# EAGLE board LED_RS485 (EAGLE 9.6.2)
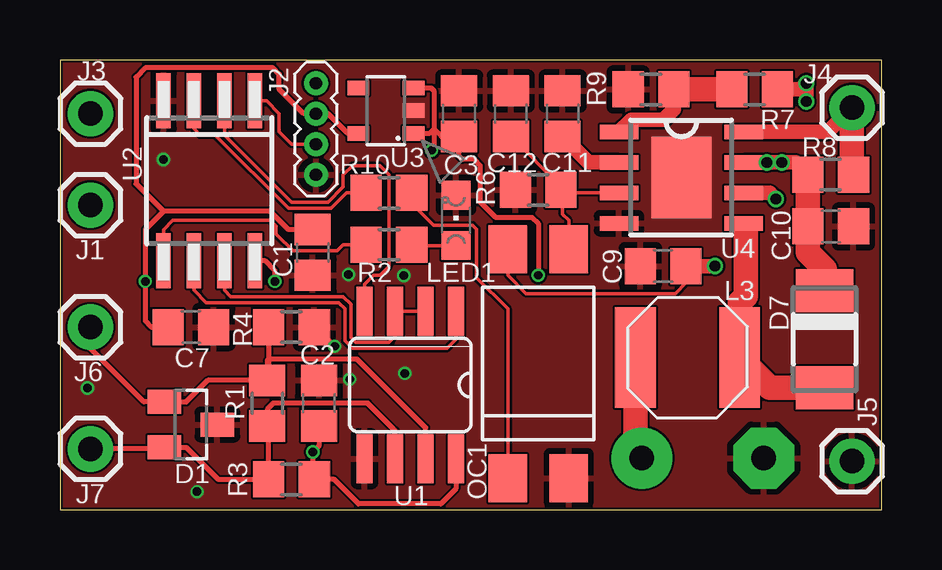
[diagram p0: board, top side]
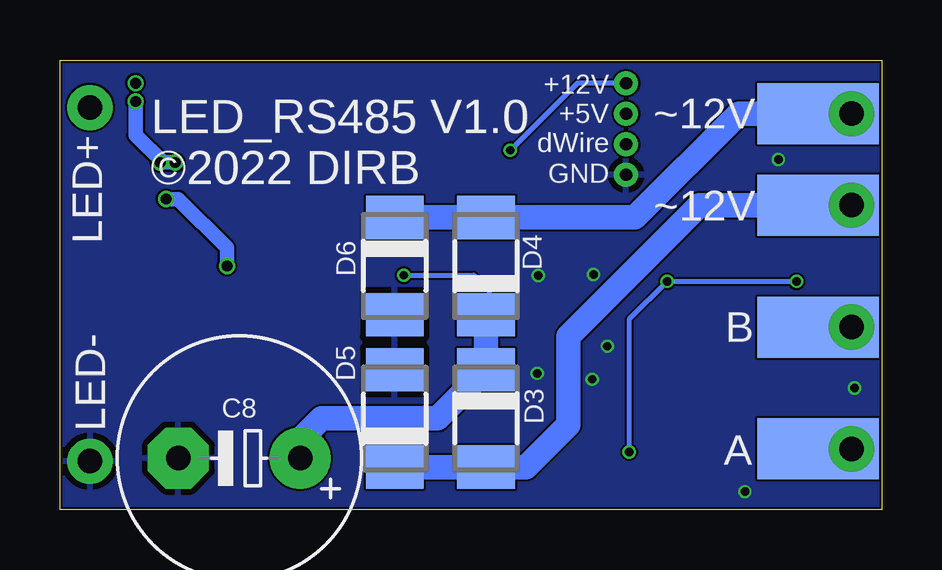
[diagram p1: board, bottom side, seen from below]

Size 34.27 x 18.75 mm. Coordinates in mm from the lower left corner, seen from the top.
Outline: 0,0 34.27,0 34.27,18.75 0,18.75 0,0
Copper layers (1*16): Top 0.035mm / dielectric 0.2mm / Bottom 0.035mm
Design rules "jlcpcb-2-layer": minimum track width 3.5mil, minimum drill 0.2mm, track to track 3.5mil, track to pad 5mil, pad to pad 5mil, via to via 5mil, smd to smd 0mil, copper to edge 0.1mm, drill to drill 5mil, minimum pad ring 4mil, minimum via ring 4mil, stop-mask expansion 3mil, vias tented up to drill 100mil, thermal gap 10mil

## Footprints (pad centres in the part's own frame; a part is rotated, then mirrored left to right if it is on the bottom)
C0805 = smd 1.3 x 1.5: 1 -0.95,0; 2 0.95,0
E5-10,5 = drill 1.016 pad 2.54: + -2.54,0 | drill 1.016 pad 2.54 octagon: - 2.54,0
SOT23 = smd 1 x 1.4: 1 -0.95,-1.1; 2 0.95,-1.1; 3 0,1.1
DO-214AC = smd 1.8 x 2.4: A 2.025,0; C -2.025,0
1X01 = drill 1.016 pad 1.88: 1 0,0
1X04_1.27MM = drill 0.508 pad 1: 1 0,0; 2 1.27,0; 3 2.54,0; 4 3.81,0
L5040S = smd 4.2 x 1.7: 1 0,2.175; 2 0,-2.175
CHIPLED_0805 = smd 1.2 x 1.2: A 0,-1.05; C 0,1.05
DIL4-SMD = smd 1.6 x 2: 1 -1.27,-4.77; 2 1.27,-4.77; 3 1.27,4.77; 4 -1.27,4.77
SMD2,54-5,08 = smd 2.54 x 5.08: 1 0,0
R0805 = smd 1.3 x 1.5: 1 -0.95,0; 2 0.95,0
SO08 = smd 0.66 x 2.032: 1 -1.905,-3.073; 2 -0.635,-3.073; 3 0.635,-3.073; 4 1.905,-3.073; 5 1.905,3.073; 6 0.635,3.073; 7 -0.635,3.073; 8 -1.905,3.073
SOIC8_EIAJ_208MIL = smd 0.6 x 2.286: 1 -1.905,-3.33; 2 -0.635,-3.33; 3 0.635,-3.33; 4 1.905,-3.33; 5 1.905,3.33; 6 0.635,3.33; 7 -0.635,3.33; 8 -1.905,3.33
SOT23-5 = smd 0.9 x 0.6: 1 -1.15,0.95; 2 -1.15,0; 3 -1.15,-0.95; 4 1.15,-0.95; 5 1.15,0.95
SOP8-EP = smd 0.6 x 1.6: 1 -1.905,-2.6; 2 -0.635,-2.6; 3 0.635,-2.6; 4 1.905,-2.6; 5 1.905,2.6; 6 0.635,2.6; 7 -0.635,2.6; 8 -1.905,2.6 | smd 3.4 x 2.5: EP 0,0

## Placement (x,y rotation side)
C1  10u  [C0805]  10.54,10.73 270 top
C2  100n  [C0805]  10.79,4.45 90 top
C3  100n  [C0805]  16.64,16.51 90 top
C7  100n  [C0805]  5.46,7.62 0 top
C8  470u/25V  [E5-10,5]  26.8,2.16 180 bottom
C9  1u  [C0805]  25.15,10.16 180 top
C10  1u  [C0805]  32.13,11.81 0 top
C11  1n  [C0805]  20.95,16.51 90 top
C12  1n  [C0805]  18.8,16.51 270 top
D1  PSM712  [SOT23]  5.46,3.56 270 top
D3  SS14  [DO-214AC]  16.51,3.81 270 bottom
D4  SS14  [DO-214AC]  16.51,10.16 90 bottom
D5  SS14  [DO-214AC]  20.32,3.81 90 bottom
D6  SS14  [DO-214AC]  20.32,10.16 270 bottom
D7  SS14  [DO-214AC]  31.88,7.11 270 top
J1  [1X01]  1.27,12.7 0 top
J2  [1X04_1.27MM]  10.67,13.97 90 top
J3  ~12V  [1X01]  1.27,16.51 0 top
J4  [1X01]  33.02,16.76 0 top
J5  [1X01]  33.02,2.03 0 top
J6  [1X01]  1.27,7.62 0 top
J7  [1X01]  1.27,2.54 0 top
L3  33uH  [L5040S]  26.16,6.35 90 top
LED1  [CHIPLED_0805]  16.51,12.06 0 top
OC1  LTV816S  [DIL4-SMD]  19.94,6.1 0 top
PAD1  ~12V  [SMD2,54-5,08]  2.67,12.7 90 bottom
PAD2  ~12V  [SMD2,54-5,08]  2.67,16.51 270 bottom
PAD5  [SMD2,54-5,08]  2.67,7.62 270 bottom
PAD6  [SMD2,54-5,08]  2.67,2.54 270 bottom
R1  120 (opt)  [R0805]  8.64,4.45 90 top
R2  1K  [R0805]  13.72,11.05 0 top
R3  360 (opt)  [R0805]  9.65,1.27 0 top
R4  360 (opt)  [R0805]  9.65,7.62 180 top
R6  4k7  [R0805]  19.94,13.34 0 top
R7  430k  [R0805]  28.96,17.53 180 top
R8  0R75  [R0805]  32.13,13.97 0 top
R9  10k  [R0805]  24.64,17.53 180 top
R10  1K  [R0805]  13.72,13.21 180 top
U1  MAX485CSA  [SO08]  14.6,5.21 180 top
U2  ATTINY85-20S  [SOIC8_EIAJ_208MIL]  6.22,13.72 180 top
U3  LP2981AIM5-5.0/NOPB  [SOT23-5]  13.59,16.64 180 top
U4  BP1808  [SOP8-EP]  25.91,13.84 270 top

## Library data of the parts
C1-C3 C7-C12 = rcl; SPICEPREFIX: C
D1 D3-D7 = diode
J1-J7 = SparkFun-Connectors
L3 = OPL_Inductor
LED1 = led
OC1 = optocoupler
PAD1 PAD2 PAD5 PAD6 = wirepad
R1-R4 R6-R10 = rcl; SPICEPREFIX: R
U1 = maxim; MPN: MAX3468CSA+; OC_FARNELL: unknown; OC_NEWARK: 76K6721
U2 = _hhn_attiny25_45_85
U3 = Regulators
U4 = BP1808

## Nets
+5V: C1.1 C2.1 C7.1 J2.3 R3.2 U1.8 U2.8 U3.5
A: D1.2 J7.1 PAD6.1 R1.1 R3.1 U1.6
B: D1.1 J6.1 PAD5.1 R1.2 R4.2 U1.7
DIR: U1.2 U1.3 U2.7
GND: C1.2 C2.2 C3.2 C7.2 C8.- C9.2 C10.2 C11.2 C12.1 D1.3 D5.A D6.A J2.1 J5.1 LED1.C OC1.2 R4.1 R6.1 R9.2 U1.5 U2.4 U3.2 U4.4 U4.EP
LED: R2.1 U2.5
N$1: C3.1 C8.+ D3.C D4.C J2.4 L3.1 U3.1 U3.3
N$6: LED1.A R2.2
N$7: R10.2 U2.3
N$10: D3.A D5.C J1.1 PAD1.1
N$11: J2.2 U2.1
N$12: C12.2 OC1.3 R6.2 U4.3
N$14: D4.A D6.C J3.1 PAD2.1
N$15: D7.A L3.2 U4.5
N$18: C9.1 OC1.4 U4.6
N$19: C11.1 U4.2
N$20: C10.1 D7.C R7.1 R8.1 U4.7
N$21: J4.1 R8.2 U4.8
N$23: R7.2 R9.1 U4.1
PWM: OC1.1 R10.1
RXD: U1.1 U2.6
TXD: U1.4 U2.2

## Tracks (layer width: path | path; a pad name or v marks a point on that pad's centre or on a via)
+5V  (via drill 0.35)
  Top 0.2: U3.5 12,15.69 11.18,16.51 J2.3 10.16,16.51 9.14,17.53 9.14,18.16 8.89,18.41 3.56,18.41 3.18,18.03 3.18,13.59 4.32,12.45 | U2.8 8.14,10.4 8.52,10.4 8.95,9.97 v8.95,9.52 | C2.1 10.79,2.67 v10.54,2.41 10.54,1.33 R3.2 11.43,1.27 12.45,0.25 15.87,0.25 16.51,0.89 U1.8 | C1.1 9.53,11.68 8.76,12.45 4.32,12.45 | 4.32,12.45 3.56,11.68 v3.56,9.52 3.56,7.87 3.81,7.62 C7.1
  Bottom 0.2: v3.56,9.52 v8.95,9.52 10.54,7.94 v10.54,2.41
A
  Top 0.2: J7.1 4.29,2.54 D1.2 5.27,2.61 6.6,1.27 R3.1 8.7,3.43 R1.1 8.64,4.19 8.89,4.45 12.83,4.45 13.97,3.3 U1.6
  Bottom 0.15: PAD6.1 J7.1
B
  Top 0.2: J6.1 1.27,6.73 3.49,4.51 D1.1 5.27,4.51 6.16,5.39 R1.2 | U1.7 15.24,3.43 12.38,6.29 8.7,6.29 8.64,6.22 R1.2 | R4.2 8.7,5.46 R1.2
  Bottom 0.15: PAD5.1 J6.1
DIR
  Top 0.15: U1.2 U1.3 13.97,7.24 13.72,6.99 12.32,6.99 12.13,7.17 12.13,8.57 11.81,8.89 7.11,8.89 6.86,9.14 U2.7
GND  (via drill 0.35)
  Top 0.2: v11.45,6.82 10.65,7.62 R4.1
  other vias: 4.32,14.61 5.71,0.76 1.14,5.08 12.08,5.44 14.37,5.69 14.33,9.76 12.03,9.81
  pour Top: 0,18.67 34.29,18.67 34.29,0 0,0 0,18.54
  pour Bottom: 0,18.67 34.29,18.67 34.29,0 0,0
LED
  Top 0.15: R2.1 11.81,11.05 11.56,10.79 9.71,10.79 9.02,11.49 9.02,11.81 8.76,12.06 4.7,12.06 4.32,11.68 U2.5
N$1  (via drill 0.35)
  Top 0.2: v19.94,9.78 19.94,11.94 19.69,12.19 18.16,12.19 17.53,12.83 17.53,14.35 17.27,14.61 16.76,14.61 16.64,14.73 C3.1 15.9,15.56 15.59,15.87 | U3.3 15.48,17.59 15.59,17.47 15.59,15.87 | 15.59,15.87 15.4,15.68 U3.1 | v15.49,14.99 15.59,15.08 15.59,15.87
  Top 1.016: C8.+ 23.99,2.43 L3.1
  Bottom 0.2: v19.94,9.78 17.02,9.78 16.38,9.14 16.38,8.26 D4.C | J2.4 12.7,17.78 v15.49,14.99
  Bottom 1.016: D4.C D3.C 18.53,3.81 23.37,3.81 24.26,2.92 C8.+
N$6
  Top 0.15: R2.2 14.7,11.02 LED1.A
N$7
  Top 0.15: R10.2 11.94,13.21 11.3,12.57 9.53,12.57 6.48,15.62 5.84,15.62 5.59,15.88 U2.3
N$10
  Bottom 0.15: PAD1.1 J1.1
  Bottom 1.016: PAD1.1 7.62,12.7 13.08,7.24 13.08,3.56 14.85,1.78 D3.A D5.C
N$11
  Top 0.15: J2.2 9.65,15.24 9.14,15.75 9.14,16.51 8.61,17.05 U2.1
N$12
  Top 0.152: U4.3 21.02,13.21 | 21.02,13.21 R6.2 20.89,13.47 C12.2 | OC1.3 21.21,12.06 20.95,12.32 20.95,13.15 21.02,13.21
N$14
  Bottom 0.15: PAD2.1 J3.1
  Bottom 1.016: D6.C D4.A 10.29,12.19 5.97,16.51 PAD2.1
N$15
  Top 0.203: 28.58,11.71 28.58,11.86 U4.5
  Top 1.016: D7.A 29.6,5.09 L3.2 28.34,8.65 28.58,8.9 28.58,11.71
N$18  (via drill 0.45)
  Top 0.152: C9.1 26.1,9.46 25.65,9.02 19.43,9.02 18.67,9.78 OC1.4
  Top 0.61: C9.1 v27.3,10.16 | U4.6 29.59,13.21 v29.84,12.95
  Bottom 0.61: v27.3,10.16 27.3,10.92 29.34,12.95 v29.84,12.95
N$19
  Top 0.61: U4.2 22.04,14.48 C11.1
N$20  (via drill 0.45)
  Top 0.61: R8.1 30.67,14.48 v30.1,14.48 v29.46,14.48 U4.7 | R7.1 30.86,17.53 v31.12,17.78 v31.12,17.02
  Top 1.016: R8.1 C10.1 31.18,10.73 31.88,10.03 D7.C
  Bottom 0.61: v31.12,17.02 31.12,15.62 29.97,14.48 v29.46,14.48
N$21
  Top 0.61: U4.8 32,15.75 J4.1
  Top 1.016: J4.1 33.02,14.03 R8.2
N$23
  Top 0.61: U4.1 23.82,16.26 25.15,16.26 25.59,16.7 R9.1
  Top 1.016: R9.1 R7.2
PWM
  Top 0.15: R10.1 14.67,12.77 15.57,11.87 17.2,11.87 17.37,11.7 17.37,9.67 18.67,8.38 OC1.1
RXD
  Top 0.15: U2.6 5.59,9.15 6.1,8.64 11.62,8.64 11.88,8.38 11.88,7.05 12.19,6.73 16.13,6.73 16.51,7.11 U1.1
TXD
  Top 0.15: U2.2 6.86,15.62 9.65,12.83 11.18,12.83 11.81,13.46 11.81,13.97 12.19,14.35 13.33,14.35 13.72,13.97 13.72,10.16 13.33,9.78 13.08,9.78 12.7,9.4 U1.4

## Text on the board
bNames: ~12V | +12V | +5V | LED+ | dWire | GND | ~12V | LED_RS485 V1.0 / ©2022 DIRB | B | LED- | A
